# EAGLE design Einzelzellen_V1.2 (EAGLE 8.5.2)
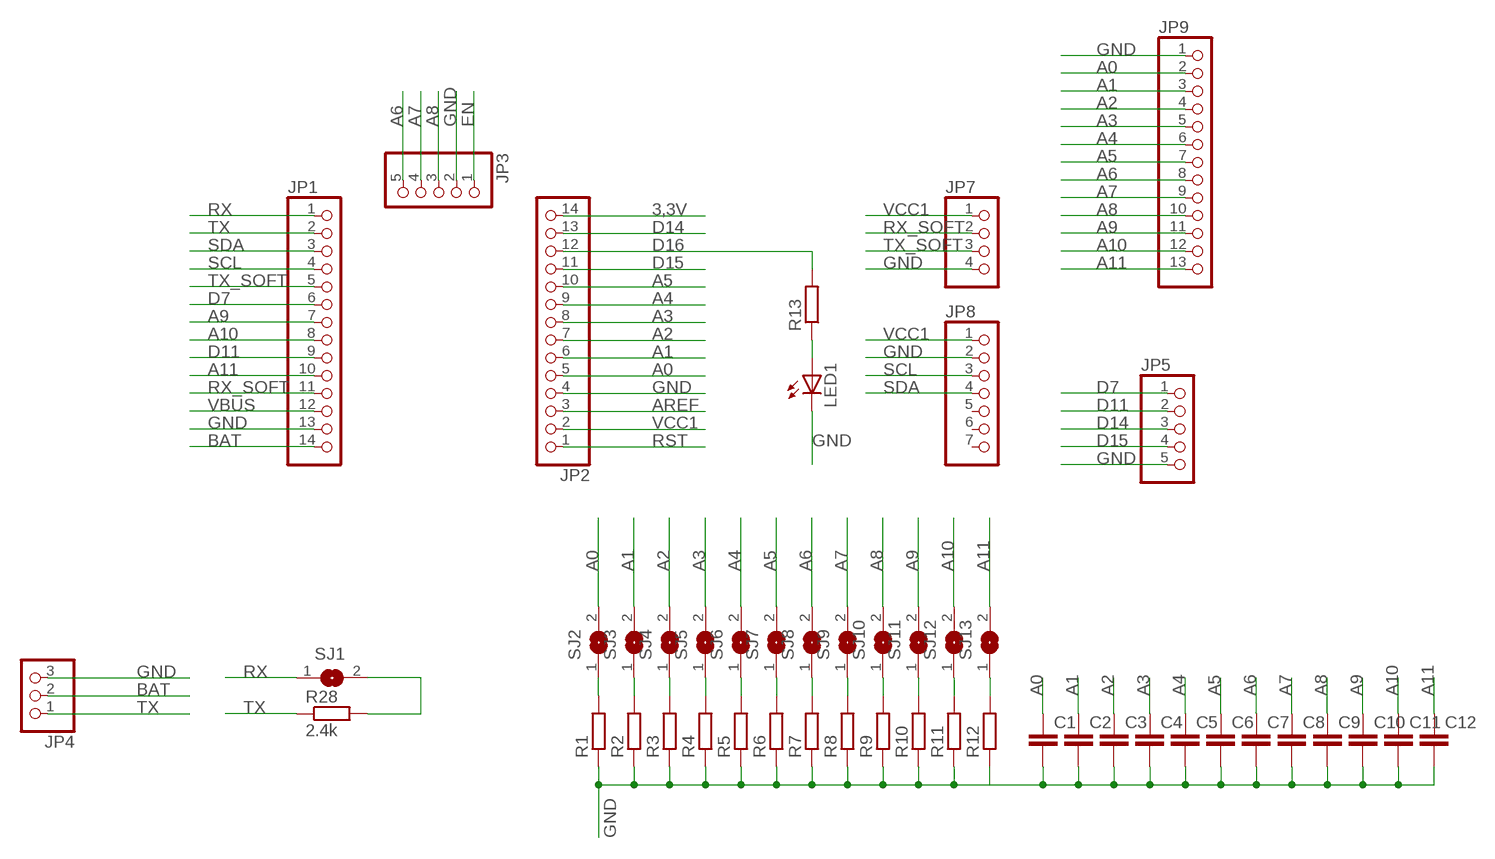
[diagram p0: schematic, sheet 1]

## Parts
C1  C-EUC0805  [C0805]
C2  C-EUC0805  [C0805]
C3  C-EUC0805  [C0805]
C4  C-EUC0805  [C0805]
C5  C-EUC0805  [C0805]
C6  C-EUC0805  [C0805]
C7  C-EUC0805  [C0805]
C8  C-EUC0805  [C0805]
C9  C-EUC0805  [C0805]
C10  C-EUC0805  [C0805]
C11  C-EUC0805  [C0805]
C12  C-EUC0805  [C0805]
JP1  PINHD-1X14  [1X14]
JP2  PINHD-1X14  [1X14]
JP3  PINHD-1X5  [1X05]
JP4  PINHD-1X3  [1X03]
JP5  PINHD-1X5  [1X05]
JP7  PINHD-1X4  [1X04]
JP8  PINHD-1X7  [1X07]
JP9  PINHD-1X13  [1X13]
LED1  LEDCHIPLED_1206  [CHIPLED_1206]
R1  R-EU_M0805  [M0805]
R2  R-EU_M0805  [M0805]
R3  R-EU_M0805  [M0805]
R4  R-EU_M0805  [M0805]
R5  R-EU_M0805  [M0805]
R6  R-EU_M0805  [M0805]
R7  R-EU_M0805  [M0805]
R8  R-EU_M0805  [M0805]
R9  R-EU_M0805  [M0805]
R10  R-EU_M0805  [M0805]
R11  R-EU_M0805  [M0805]
R12  R-EU_M0805  [M0805]
R13  R-EU_M0805  [M0805]
R28  2.4k  R-EU_M0805  [M0805]
SJ1  SJ  [SJ]
SJ2  SJ  [SJ]
SJ3  SJ  [SJ]
SJ4  SJ  [SJ]
SJ5  SJ  [SJ]
SJ6  SJ  [SJ]
SJ7  SJ  [SJ]
SJ8  SJ  [SJ]
SJ9  SJ  [SJ]
SJ10  SJ  [SJ]
SJ11  SJ  [SJ]
SJ12  SJ  [SJ]
SJ13  SJ  [SJ]

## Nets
3,3V: JP2.14
A0: C1.1 JP2.5 JP9.2 SJ2.2
A1: C2.1 JP2.6 JP9.3 SJ3.2
A2: C3.1 JP2.7 JP9.4 SJ4.2
A3: C4.1 JP2.8 JP9.5 SJ5.2
A4: C5.1 JP2.9 JP9.6 SJ6.2
A5: C6.1 JP2.10 JP9.7 SJ7.2
A6: C7.1 JP3.5 JP9.8 SJ8.2
A7: C8.1 JP3.4 JP9.9 SJ9.2
A8: C9.1 JP3.3 JP9.10 SJ10.2
A9: C10.1 JP1.7 JP9.11 SJ11.2
A10: C11.1 JP1.8 JP9.12 SJ12.2
A11: C12.1 JP1.10 JP9.13 SJ13.2
AREF: JP2.3
BAT [BAT]: JP1.14 JP4.2
D7: JP1.6 JP5.1
D11: JP1.9 JP5.2
D14: JP2.13 JP5.3
D15: JP2.11 JP5.4
D16: JP2.12 R13.2
EN: JP3.1
GND [GND]: C1.2 C2.2 C3.2 C4.2 C5.2 C6.2 C7.2 C8.2 C9.2 C10.2 C11.2 C12.2 JP1.13 JP2.4 JP3.2 JP4.3 JP5.5 JP7.4 JP8.2 JP9.1 LED1.C R1.1 R2.1 R3.1 R4.1 R5.1 R6.1 R7.1 R8.1 R9.1 R10.1 R11.1 R12.1
N$1: R28.2 SJ1.2
N$2: R1.2 SJ2.1
N$3: R2.2 SJ3.1
N$4: R3.2 SJ4.1
N$5: R4.2 SJ5.1
N$6: R5.2 SJ6.1
N$7: R6.2 SJ7.1
N$8: R7.2 SJ8.1
N$9: R8.2 SJ9.1
N$10: R9.2 SJ10.1
N$11: R10.2 SJ11.1
N$12: R11.2 SJ12.1
N$13: R12.2 SJ13.1
N$14: LED1.A R13.1
RST: JP2.1
RX: JP1.1 SJ1.1
RX_SOFT: JP1.11 JP7.2
SCL: JP1.4 JP8.3
SDA: JP1.3 JP8.4
TX: JP1.2 JP4.1 R28.1
TX_SOFT: JP1.5 JP7.3
VBUS: JP1.12
VCC1 [VCC1]: JP2.2 JP7.1 JP8.1
Unconnected: JP8.5 JP8.6 JP8.7

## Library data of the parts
C1-C12 = resistor:C-EU: CAPACITOR, European symbol
JP1 JP2 = pinhead:PINHD-1X14: PIN HEADER
JP3 JP5 = pinhead:PINHD-1X5: PIN HEADER
JP4 = pinhead:PINHD-1X3: PIN HEADER
JP7 = pinhead:PINHD-1X4: PIN HEADER
JP8 = pinhead:PINHD-1X7: PIN HEADER
JP9 = pinhead:PINHD-1X13: PIN HEADER
LED1 = led:LED: LED
R1-R13 R28 = resistor:R-EU_: RESISTOR, European symbol
SJ1-SJ13 = jumper:SJ: SMD solder JUMPER

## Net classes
1 VCC: width 0.305 mm
2 GND: width 0.305 mm
3 VCC1: width 0.305 mm
4 BAT: width 0.305 mm

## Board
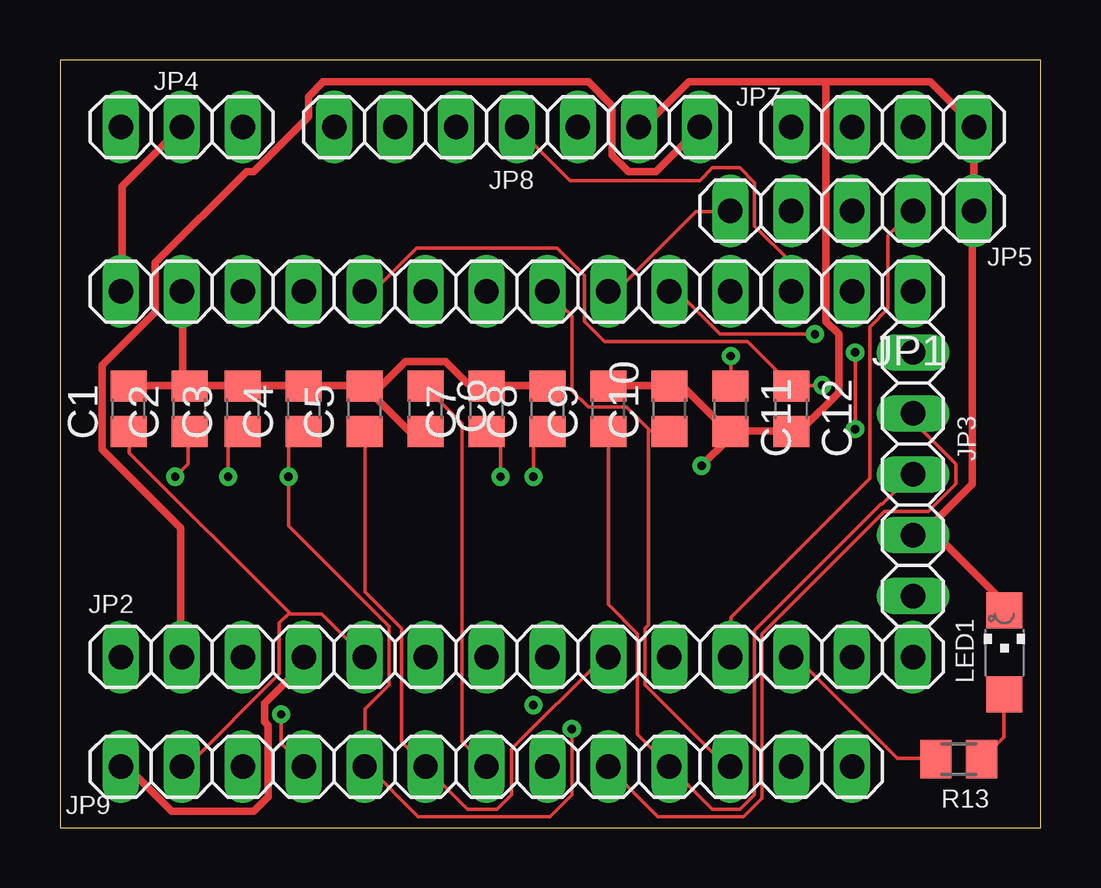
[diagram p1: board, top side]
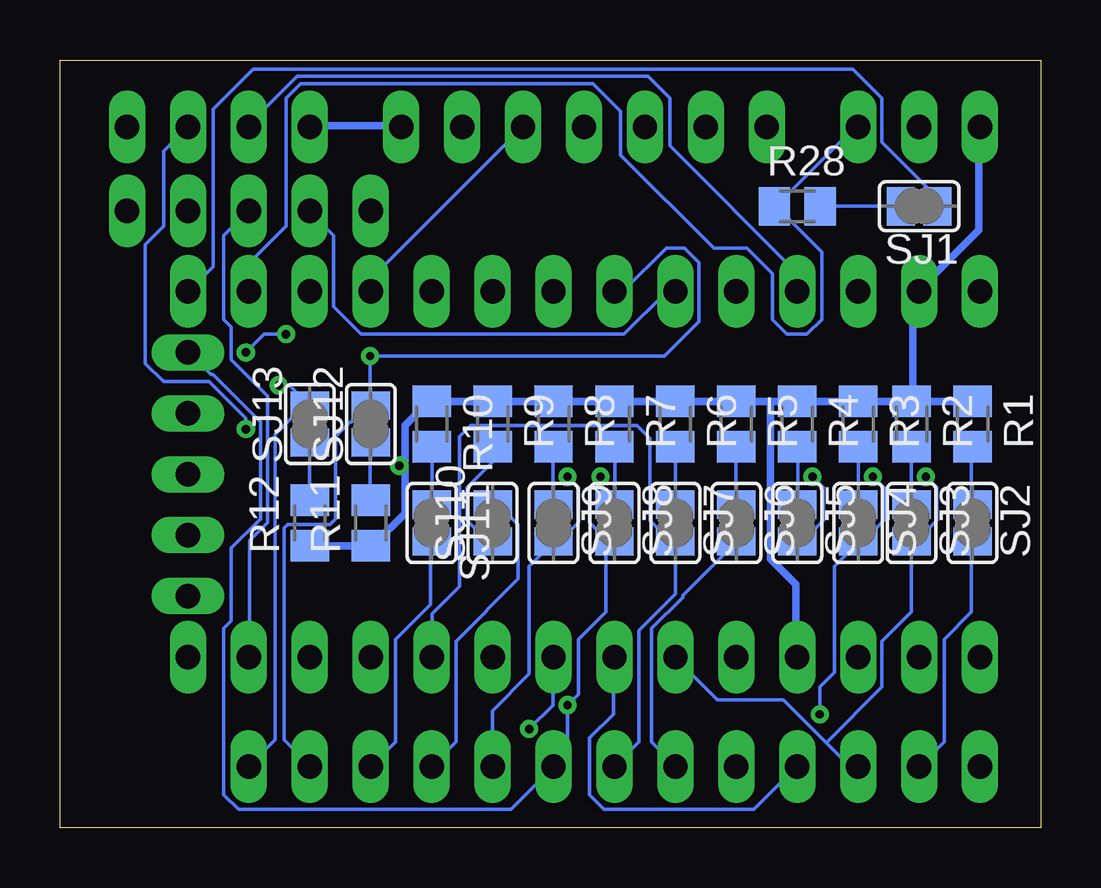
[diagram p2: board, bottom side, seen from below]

Size 40.89 x 32 mm. Coordinates in mm from the lower left corner, seen from the top.
Outline: 0,0 40.89,0 40.89,32 0,32 0,0
Copper layers (1*16): Top 0.035mm / dielectric 1.5mm / Bottom 0.035mm
Design rules "default *": minimum track width 6mil, minimum drill 0.35mm, track to track 6mil, track to pad 6mil, pad to pad 6mil, via to via 6mil, smd to smd 6mil, copper to edge 2mil, drill to drill 6mil, minimum pad ring 10mil, minimum via ring 8mil, stop-mask expansion 4mil, vias tented up to drill 0mil, thermal gap 10mil

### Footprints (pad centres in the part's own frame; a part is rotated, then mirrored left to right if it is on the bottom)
C0805 = smd 1.3 x 1.5: 1 -0.95,0; 2 0.95,0
1X14 = drill 1.016 long: 1 -16.51,0; 2 -13.97,0; 3 -11.43,0; 4 -8.89,0; 5 -6.35,0; 6 -3.81,0; 7 -1.27,0; 8 1.27,0; 9 3.81,0; 10 6.35,0; 11 8.89,0; 12 11.43,0; 13 13.97,0; 14 16.51,0
1X05 = drill 1.016 long: 1 -5.08,0; 2 -2.54,0; 3 0,0; 4 2.54,0; 5 5.08,0
1X03 = drill 1.016 long: 1 -2.54,0; 2 0,0; 3 2.54,0
1X04 = drill 1.016 long: 1 -3.81,0; 2 -1.27,0; 3 1.27,0; 4 3.81,0
1X07 = drill 1.016 long: 1 -7.62,0; 2 -5.08,0; 3 -2.54,0; 4 0,0; 5 2.54,0; 6 5.08,0; 7 7.62,0
1X13 = drill 1.016 long: 1 -15.24,0; 2 -12.7,0; 3 -10.16,0; 4 -7.62,0; 5 -5.08,0; 6 -2.54,0; 7 0,0; 8 2.54,0; 9 5.08,0; 10 7.62,0; 11 10.16,0; 12 12.7,0; 13 15.24,0
CHIPLED_1206 = smd 1.5 x 1.5: A 0,-1.75; C 0,1.75
M0805 = smd 1.3 x 1.6: 1 -0.95,0; 2 0.95,0
SJ = smd 1.168 x 1.6: 1 -0.762,0; 2 0.762,0

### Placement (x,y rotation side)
C1  2.86,17.46 90 top
C2  5.4,17.46 90 top
C3  7.62,17.46 90 top
C4  10.16,17.46 90 top
C5  12.7,17.46 90 top
C6  15.24,17.46 270 top
C7  17.78,17.46 90 top
C8  20.32,17.46 90 top
C9  22.86,17.46 90 top
C10  25.4,17.46 90 top
C11  27.94,17.46 270 top
C12  30.48,17.46 270 top
JP1  19.05,22.35 180 top
JP2  19.05,7.11 0 top
JP3  35.56,14.73 90 top
JP4  5.08,29.21 180 top
JP5  33.02,25.72 0 top
JP7  34.29,29.21 0 top
JP8  19.05,29.21 180 top
JP9  17.78,2.54 0 top
LED1  39.37,7.3 0 top
R1  2.86,16.83 270 bottom
R2  5.4,16.83 270 bottom
R3  7.62,16.83 270 bottom
R4  10.16,16.83 270 bottom
R5  12.7,16.83 270 bottom
R6  15.24,16.83 270 bottom
R7  17.78,16.83 270 bottom
R8  20.32,16.83 270 bottom
R9  22.86,16.83 270 bottom
R10  25.4,16.83 270 bottom
R11  27.94,12.7 90 bottom
R12  30.48,12.7 90 bottom
R13  37.47,2.86 180 top
R28  10.16,25.91 0 bottom
SJ1  5.08,25.91 180 bottom
SJ2  2.86,12.7 270 bottom
SJ3  5.4,12.7 270 bottom
SJ4  7.62,12.7 270 bottom
SJ5  10.16,12.7 270 bottom
SJ6  12.7,12.7 270 bottom
SJ7  15.24,12.7 270 bottom
SJ8  17.78,12.7 270 bottom
SJ9  20.32,12.7 270 bottom
SJ10  22.86,12.7 90 bottom
SJ11  25.4,12.7 270 bottom
SJ12  27.94,16.83 90 bottom
SJ13  30.48,16.83 90 bottom

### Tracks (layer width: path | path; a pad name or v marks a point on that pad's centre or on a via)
A0
  Top 0.152: 9.56,8.95 9.6,8.91 10.9,8.91 JP2.5 | 9.56,8.95 2.9,15.62 2.9,16.46 C1.1 | 9.56,8.95 9.14,8.53 9.14,6.4 5.33,2.59 5.11,2.59 JP9.2
  Bottom 0.152: JP9.2 4.04,3.58 4.04,7.85 2.9,8.99 2.9,11.89 SJ2.2
A1  (via drill 0.35)
  Top 0.152: v4.8,14.63 5.33,15.16 5.33,16.46 C2.1
  Bottom 0.152: v4.8,14.63 4.34,14.17 4.34,12.8 5.18,11.96 5.33,11.96 SJ3.2 5.41,11.89 5.41,8.99 6.63,7.77 6.63,5.87 8.95,3.54 | 8.95,3.54 10.74,5.33 13.49,5.33 15.24,7.09 JP2.6 | 8.95,3.54 8,2.59 7.62,2.59 JP9.3
A2  (via drill 0.35)
  Top 0.152: v9.22,4.72 9.22,3.5 10.13,2.59 JP9.4 | v7.01,14.63 7.01,15.85 7.62,16.46 C3.1
  Bottom 0.152: v7.01,14.63 6.55,14.17 6.55,12.8 7.39,11.96 7.62,11.96 SJ4.2 7.62,11.89 8.61,10.9 8.61,6.48 9.22,5.87 v9.22,4.72 | JP2.7 17.83,7.09 17.83,4.72 18.82,3.73 18.82,1.37 18.21,0.76 11.96,0.76 10.21,2.52 JP9.4
A3  (via drill 0.35)
  Top 0.152: C4.1 10.13,16.46 9.53,15.85 v9.53,14.63 9.53,12.57 13.72,8.38 13.72,5.94 12.72,4.95 12.72,2.59 JP9.5 12.8,2.59 14.94,0.46 20.42,0.46 21.34,1.37 v21.34,4.12
  Bottom 0.152: v9.53,14.63 9.07,14.17 9.07,12.8 9.91,11.96 10.13,11.96 SJ5.2 | v21.34,4.12 20.34,5.11 20.34,7.09 JP2.8
A4
  Top 0.152: C5.1 12.72,16.46 12.72,9.83 14.25,8.31 14.25,3.58 15.24,2.59 JP9.6 15.24,2.52 16.99,0.76 18.21,0.76 18.82,1.37 18.82,3.28 22.63,7.09 22.86,7.09 JP2.9
  Bottom 0.152: SJ6.2 12.72,11.89 14.94,9.68 14.94,9.6 16.23,8.31 16.23,3.58 15.24,2.59 JP9.6
A5
  Top 0.152: C6.1 15.24,18.36 16.76,16.84 16.76,3.58 17.75,2.59 JP9.7
  Bottom 0.152: JP9.7 17.75,2.59 16.76,3.58 16.76,8.23 15.24,9.75 SJ7.2 15.24,11.96 15.47,11.96 16.31,12.8 16.31,16.23 16.84,16.76 23.77,16.76 24.23,16.31 24.23,10.06 25.38,8.91 25.38,7.16 JP2.10
A6  (via drill 0.35)
  Top 0.152: v18.36,14.63 18.36,15.93 17.83,16.46 C7.1
  Bottom 0.152: v18.36,14.63 18.82,14.17 18.82,12.72 18.06,11.96 17.83,11.96 SJ8.2 18.14,11.96 18.14,8.99 19.28,7.85 19.28,5.56 v19.74,5.11 19.74,3.12 JP9.8 22.1,0.76 33.45,0.76 34.06,1.37 34.06,8.31 33.76,8.61 33.76,11.66 32.54,12.88 32.54,16.92 34.52,18.9 34.59,18.9 35.51,19.81 JP3.5
A7  (via drill 0.35)
  Top 0.152: v19.74,14.63 19.74,15.93 20.27,16.46 C8.1 | JP3.4 35.59,17.22 35.59,16.92 37.34,15.16 37.34,14.33 36.2,13.18 34.37,13.18 29.26,8.08 29.26,1.22 28.5,0.46 24.92,0.46 22.86,2.52 JP9.9
  Bottom 0.152: v19.74,14.63 19.28,14.17 19.28,12.72 20.04,11.96 20.27,11.96 SJ9.2 20.34,11.89 21.34,10.9 21.34,6.4 22.86,4.88 JP9.9
A8
  Top 0.152: C9.1 22.86,9.3 24.08,8.08 24.08,3.89 25.38,2.59 JP9.10 25.45,2.52 27.2,0.76 28.35,0.76 28.96,1.37 28.96,8.23 34.21,13.49 34.29,13.49 35.51,14.71 JP3.3
  Bottom 0.152: SJ10.2 22.86,13.41 22.55,13.41 21.79,12.65 21.79,10.36 24.38,7.77 24.38,3.58 25.38,2.59 JP9.10
A9
  Top 0.152: 24.57,16.57 23.62,17.53 22.02,17.53 21.34,18.21 21.34,21.34 JP1.7 | 24.57,16.57 24.61,16.54 25.38,16.54 C10.1 | 24.57,16.57 24.54,16.54 24.54,8.46 24.38,8.31 24.38,5.94 27.74,2.59 27.89,2.59 JP9.11
  Bottom 0.152: JP9.11 26.9,3.58 26.9,7.85 25.45,9.3 25.45,11.89 SJ11.2
A10  (via drill 0.35)
  Top 0.152: v27.96,19.66 27.96,18.44 C11.1
  Bottom 0.152: JP9.12 30.48,2.59 31.55,3.66 31.55,12.5 31.39,12.65 29.64,12.65 29.41,12.88 29.41,16.31 28.8,16.92 28.73,16.92 28.04,17.6 SJ12.2 27.96,17.6 v27.96,19.66 15.7,19.66 14.25,21.11 14.25,23.55 14.86,24.16 15.62,24.16 17.37,22.4 17.75,22.4 JP1.8
A11  (via drill 0.35)
  Top 0.152: v31.77,18.44 30.48,18.44 | 30.48,18.44 28.65,20.27 22.71,20.27 21.87,21.11 21.87,23.01 20.73,24.16 14.86,24.16 13.11,22.4 12.72,22.4 JP1.10 | 30.48,18.44 C12.1
  Bottom 0.152: v31.77,18.44 31.32,18.44 30.48,17.6 SJ13.2 30.63,17.68 31.93,16.38 31.93,3.66 32.99,2.59 JP9.13
BAT
  Top 0.305: JP1.14 2.59,22.4 2.59,26.75 5.03,29.18 JP4.2
D7
  Top 0.152: JP1.6 22.86,22.4 23.24,22.4 26.52,25.68 27.89,25.68 JP5.1
D11
  Bottom 0.152: JP1.9 15.24,22.33 15.62,22.33 17.37,20.57 28.35,20.57 29.49,21.72 29.49,24.69 30.48,25.68 JP5.2
D14
  Bottom 0.152: JP2.13 32.99,7.16 32.99,11.96 32.23,12.72 32.23,17.98 33.76,19.51 33.76,20.88 34.06,21.18 34.06,24.69 33.07,25.68 JP5.3
D15
  Top 0.152: JP2.11 27.96,7.16 27.96,8.76 33.76,14.55 33.76,20.88 34.52,21.64 34.52,24.69 35.51,25.68 JP5.4
D16
  Top 0.152: R13.2 36.5,2.9 34.9,2.9 30.71,7.09 30.48,7.09 JP2.12
GND  (via drill 0.35)
  Top 0.305: C1.2 2.9,18.44 5.33,18.44 C2.2 | 7.7,18.44 C3.2 | 10.06,18.44 C4.2 | C9.2 22.86,18.44 25.38,18.44 C10.2 25.53,18.36 25.98,18.36 27.81,16.54 C11.2 | C11.2 27.96,16.54 30.48,16.54 C12.2 30.56,16.61 30.94,16.61 32.46,18.14 32.46,20.57 31.93,21.11 31.93,31.09 | LED1.C 39.66,9.07 36.54,12.19 JP3.2 35.81,12.12 38.02,14.33 38.02,25.6 JP5.5 JP7.4 38.1,29.26 36.27,31.09 31.93,31.09 | 31.93,31.09 26.21,31.09 24.38,29.26 24.16,29.26 JP8.2 | C8.2 20.27,18.44 17.83,18.44 C7.2 17.68,18.52 16.99,18.52 16.08,19.43 14.4,19.43 13.11,18.14 C5.2 | C3.2 7.47,18.44 5.49,18.44 C2.2 | C3.2 7.85,18.44 9.91,18.44 C4.2 | C5.2 12.65,18.44 10.29,18.44 C4.2 | C6.2 15.24,16.54 14.55,16.54 12.8,18.29 C5.2 | JP1.13 5.11,22.33 5.11,18.52 C2.2 | JP9.1 2.59,2.52 2.82,2.52 4.65,0.69 8.08,0.69 8.69,1.29 8.69,4.27 8.53,4.42 8.53,5.18 10.13,6.78 10.13,7.09 JP2.4 | v26.75,15.09 27.81,16.15 27.81,16.38 C11.2
  Bottom 0.305: R12.1 30.48,11.73 27.96,11.73 R11.1 27.81,11.81 26.52,13.11 26.52,15.09 | 25.38,17.75 R10.1 | 22.94,17.75 R9.1 | JP1.13 5.33,22.1 | 5.33,17.91 R2.1 | JP4.3 2.59,29.18 2.59,24.92 5.03,22.48 JP1.13 | R9.1 22.71,17.75 20.34,17.75 R8.1 20.19,17.75 17.91,17.75 R7.1 17.75,17.75 15.32,17.75 R6.1 15.24,17.75 12.8,17.75 R5.1 12.65,17.75 11.28,17.75 | R10.1 25.22,17.75 23.09,17.75 R9.1 | 26.52,15.09 26.52,16.76 25.53,17.75 R10.1 | R1.1 2.9,17.75 5.26,17.75 R2.1 | R2.1 5.49,17.75 7.62,17.75 R3.1 7.7,17.75 10.13,17.75 R4.1 10.29,17.75 11.28,17.75 | 11.28,17.75 11.28,11.2 10.21,10.13 10.21,7.16 JP2.4 | JP1.13 5.33,22.02 5.33,18.06 R2.1 | 26.52,15.09 v26.75,15.09
N$1
  Bottom 0.152: SJ1.2 R28.2
N$2
  Bottom 0.152: 2.9,15.85 R1.2 2.9,15.77 2.9,13.56 SJ2.1 2.9,13.49
N$3
  Bottom 0.152: R2.2 5.41,15.85 5.41,13.49 SJ3.1
N$4
  Bottom 0.152: SJ4.1 R3.2
N$5
  Bottom 0.152: R4.2 10.13,15.85 10.13,13.49 SJ5.1
N$6
  Bottom 0.152: R5.2 12.72,15.85 12.72,13.49 SJ6.1
N$7
  Bottom 0.152: SJ7.1 R6.2
N$8
  Bottom 0.152: R7.2 17.75,15.85 17.75,13.49 SJ8.1
N$9
  Bottom 0.152: R8.2 20.34,15.85 20.34,13.49 SJ9.1
N$10
  Bottom 0.152: R9.2 22.86,15.24 23.93,14.17 23.93,12.8 23.09,11.96 22.86,11.96 SJ10.1
N$11
  Bottom 0.152: R10.2 25.38,15.85 25.38,13.49 SJ11.1
N$12
  Bottom 0.152: 27.96,13.72 R11.2 27.96,13.79 27.96,15.93 SJ12.1 27.96,16
N$13
  Bottom 0.152: SJ13.1 R12.2
N$14
  Top 0.152: LED1.A 39.34,6.12 39.34,3.76 38.48,2.9 R13.1
RX
  Bottom 0.152: JP1.1 34.52,23.39 34.52,29.95 32.84,31.62 7.85,31.62 6.63,30.4 6.63,28.57 4.34,26.29 4.34,25.91 SJ1.1
RX_SOFT
  Bottom 0.152: JP1.11 10.21,22.4 10.21,23.16 15.47,28.42 15.47,30.4 16.38,31.32 31.01,31.32 33.07,29.26 JP7.2
SCL
  Bottom 0.152: JP1.4 27.89,22.4 27.89,22.94 21.64,29.18 JP8.3
SDA
  Top 0.152: JP1.3 30.48,23.55 28.96,25.07 28.96,26.9 28.35,27.51 27.2,27.51 26.67,26.98 21.26,26.98 19.05,29.18 JP8.4
TX
  Bottom 0.152: 11.05,25.91 7.77,29.18 7.62,29.18 JP4.1 | 11.05,25.91 9.14,24 9.14,21.18 9.75,20.57 10.59,20.57 11.2,21.18 11.2,23.09 12.27,24.16 13.64,24.16 17.53,28.04 17.53,29.87 18.67,31.01 30.86,31.01 31.47,30.4 31.47,25.07 32.99,23.55 32.99,22.4 JP1.2 | 11.05,25.91 R28.1
TX_SOFT  (via drill 0.35)
  Top 0.152: v31.47,20.57 27.51,20.57 25.76,22.33 25.45,22.33 JP1.5 | v33.15,16.61 v33.15,19.81
  Bottom 0.152: v31.47,20.57 32.38,20.57 v33.15,19.81 | v33.15,16.61 33.15,17.07 34.67,18.59 36.58,18.59 37.34,19.36 37.34,24.31 36.58,25.07 36.58,28.19 JP7.3
VCC1
  Top 0.305: JP2.2 5.03,7.16 5.03,12.5 1.75,15.77 1.75,19.28 3.96,21.49 3.96,23.55 7.77,27.36 8.08,27.36 10.36,29.64 10.36,30.48 10.97,31.09 22.02,31.09 23.01,30.1 23.01,28.04 23.7,27.36 24.84,27.36 26.67,29.18 JP8.1
  Bottom 0.305: 30.48,29.26 JP7.1 30.4,29.26 26.75,29.26 JP8.1 26.67,29.26

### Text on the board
tOrigins: SDA | SCL | GND | VCC | VCC | RX | TX | GND | GND | VCC | Sig | D7 | D11 | D14 | D15 | GND | GND | D15 | D11 | D7 | D5 | MULI 1.2 03.01.2023 | GND | 1 | 2 | 3 | 4 | 5 | 6 | 7 | 8 | 9 | 10 | 11 | 12 | JP9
